PROGRAM MAIN
VAR
	Ax:Axis_PTP_Ex2;
	
	bPowerOn: BOOL;
	bPowerOff: BOOL;
	bMove: BOOL;
	bStop: BOOL;
	
	DrvIn:ST_DrvIn;
	PARA:ST_AxisPara;
	Status:ST_AxisStatus;
	
	bReady: BOOL;
	bReset: BOOL;
	bHome: BOOL;
END_VAR

;
PARA.MoveVelo:=1000;		//准备运动的速度

Ax(DrvIn:=DrvIn , PARA:=PARA ); //调用FB实例

// 以下为4个Method的引用，实现轴的使能和启停
IF bPowerOn THEN	
	Ax.M_PowerOn();	
END_IF

IF bPowerOff THEN
	Ax.M_PowerOff();	
END_IF

Ax.M_MoveVel(Execute:=bMove );
Ax.M_Stop(Execute:=bStop );

// 刷新轴的状态
Status:=Ax.P_Status;


PARA.MoveVelo:=1000;		//准备运动的速度

Ax(DrvIn:=DrvIn , PARA:=PARA ); //调用FB实例

IF bPowerOn THEN
	Ax.M_PowerOn();	
END_IF

IF bPowerOff THEN
	Ax.M_PowerOff();	
END_IF


Ax.M_MoveVel(Execute:=bMove );
Ax.M_Stop(Execute:=bStop );
Status:=Ax.P_Status;

Ax.M_Cyclic();
Ax.M_Reset(Execute:=bReset );
Ax.M_Home(Execute:=bHome );

END_PROGRAM
